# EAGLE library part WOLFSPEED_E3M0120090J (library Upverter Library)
Silicon Carbide Power MOSFET E-Series Automotive N-Channel 22A 83W RDS(on) 120mohm
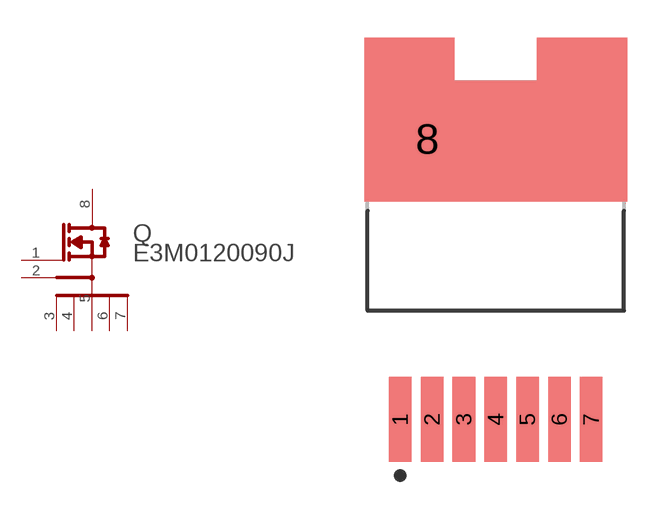
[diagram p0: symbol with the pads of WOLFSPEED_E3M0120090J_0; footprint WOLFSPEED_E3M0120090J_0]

Designator prefix Q

## WOLFSPEED_E3M0120090JWOLFSPEED_E3M0120090J_0_0 (MF: Wolfspeed; MPN: E3M0120090J; automotive: Yes; automotive_grade: Grade 0; centroid_not_specified: Yes; continuous_drain_current: 22A; datasheet: https://assets.wolfspeed.com/uploads/2021/05/E3M0120090J.pdf; depletion_mode: False; device_class_L1: Discrete Semiconductors; device_class_L2: Transistors; device_class_L3: MOSFETs; digikey_description: 900V 120M AUTOMOTIVE SIC MOSFET; digikey_part_number: 1697-E3M0120090J-ND; drain_to_source_breakdown_voltage: 900V; drain_to_source_resistance: 120mΩ; drain_to_source_voltage: 900V; footprint_variant_name_0: Recommended_Land_Pattern; gate_charge_at_vgs: 18nC @ 15V; gate_to_source_voltage: 19V; height: 4.82mm; input_capacitace_at_vds: 414pF @ 600V; lead_free: Yes; max_junction_temp: +150°C; mfg_package_ident: TO-263-7; mfg_package_ident_component_id: d2de6d38281de76c; mfg_package_ident_date: 0; mfg_package_ident_rev: 0; mouser_part_number: 941-E3M0120090J; number_of_N_channels: 1; number_of_channels: 1; package: TO-263-7; power_dissipation: 83W; prefix: Q; pulse_drain_current: 50A; reverse_recovery_charge: 72nC; reverse_recovery_time: 10ns; rohs: Yes; rthja_max: 40°C/W; standoff_height: 0mm; technology: SiC; temperature_range_high: +150°C; temperature_range_low: -55°C; threshold_vgs_max: 3.5V; threshold_vgs_min: 1.8V; transconductance: 8.9S; turn_off_delay_time: 13ns; turn_on_delay_time: 5ns; typ_forward_diode_voltage: 4.8V; verification_version: 0.0.0.3)  [WOLFSPEED_E3M0120090J_0]
1  GATE  pas
2  DRIVER_SOURCE  pas
3  1_POWER_SOURCE  pas
4  2_POWER_SOURCE  pas
5  3_POWER_SOURCE  pas
6  4_POWER_SOURCE  pas
7  5_POWER_SOURCE  pas
8  DRAIN  pas

## Footprint WOLFSPEED_E3M0120090J_0 (pad centres in mm)
Silicon Carbide Power MOSFET E-Series Automotive N-Channel 22A 83W RDS(on) 120mohm
smd 0.9 x 3.4: 1 -3.81,-6.764; 2 -2.54,-6.764; 3 -1.27,-6.764; 4 0,-6.764; 5 1.27,-6.764; 6 2.54,-6.764; 7 3.81,-6.764
smd 4.505 x 4.505: 8 -2.737,4.429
